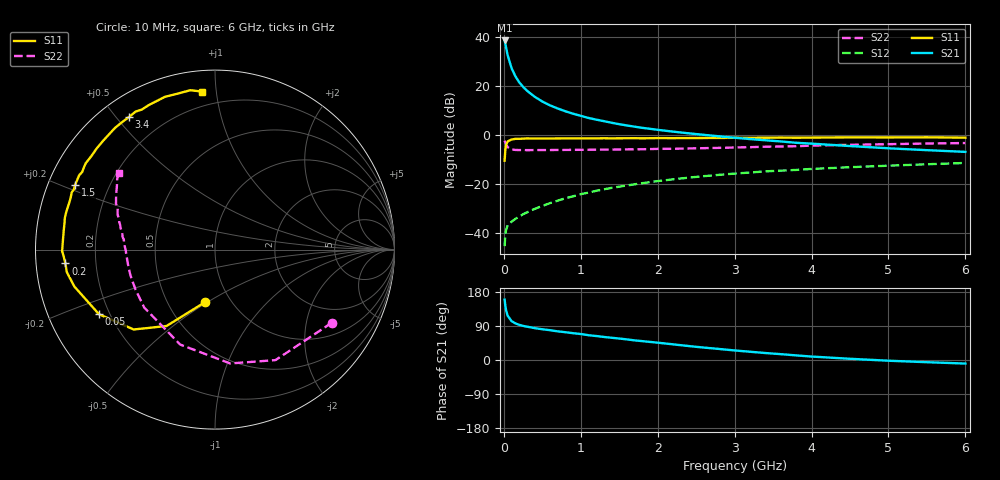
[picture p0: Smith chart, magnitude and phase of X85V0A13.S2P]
! SIEMENS Small Signal Semiconductors
! BFP136W
! Si NPN RF Bipolar Junction Transistor in SOT343
! VCE = 5 V  IC = 130 mA
! Common Emitter S-Parameters:  September  1994
# GHz  S  MA  R  50
!  f  S11  S21  S12  S22
! GHz  MAG  ANG  MAG  ANG  MAG  ANG  MAG  ANG
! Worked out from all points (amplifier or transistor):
!   40 points, 10 MHz to 6 GHz, reference 50 ohm
!   highest |S21| = 38.7 dB at 10 MHz (marker M1)
!   |S21| within 3 dB of that: start of sweep to 29.86 MHz
!   unconditionally stable (mu >= 1): 495.4 MHz to 2.976 GHz
!   at 200 MHz: K = 0.71, MSG = 27.5 dB, |S12| = -33.4 dB
!   at 1.5 GHz: K = 1.10, MAG = 10.9 dB, |S12| = -21.1 dB
!   at 6 GHz: K = 0.97, MSG = 2.3 dB, |S12| = -11.4 dB
!   S11 on the Smith chart (normalised r, x): 10 MHz: 0.76, -0.49; 50 MHz: 0.16, -0.25; 200 MHz: 0.09, -0.05; 1.5 GHz: 0.08, +0.22; 3.4 GHz: 0.08, +0.54; 6 GHz: 0.11, +0.91
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0.01  0.2988 -100.9  86.44 159.3  0.0053 67.9  0.7682 -32.0
0.02  0.5042 -122.4  73.26 142.2  0.0094 54.5  0.7019 -61.3
0.03  0.6351 -135.5  61.04 130.4  0.0115 48.6  0.64 -82.4
0.05  0.74 -150.9  42.98 116.6  0.0142 38.1  0.5635 -110.1
0.1  0.8102 -165.3  23.55 102.7  0.0168 37.5  0.5097 -140.7
0.15  0.8353 -171.4  15.98 96.6  0.0192 40.6  0.4956 -153.2
0.2  0.8368 -174.7  12.01 92.8  0.0215 42.7  0.4925 -159.8
0.25  0.8446 -177.6  9.676 90.0  0.0239 45.9  0.4922 -164.2
0.3  0.8518 -179.4  8.094 88.0  0.0261 48.4  0.4909 -167.0
0.4  0.849 177.0  6.098 84.2  0.0307 52.8  0.4919 -170.9
0.5  0.8488 174.3  4.859 81.1  0.0353 55.5  0.4926 -173.6
0.6  0.8498 172.3  4.055 78.7  0.0403 57.5  0.4933 -175.4
0.7  0.8517 169.8  3.496 75.6  0.0453 59.4  0.495 -176.7
0.9  0.8547 166.2  2.735 70.8  0.0557 60.6  0.4968 -179.2
1.1  0.8531 161.9  2.238 65.4  0.0663 61.2  0.5001 179.2
1.5  0.8585 155.3  1.667 56.6  0.0877 60.3  0.5056 176.0
2.2  0.8637 142.9  1.174 41.3  0.1238 55.2  0.523 170.6
3.2  0.8788 126.1  0.827 21.8  0.1708 45.5  0.5643 161.9
3.4  0.8804 123.0  0.782 18.4  0.1804 43.5  0.5767 160.2
4.5  0.8957 108.1  0.595 3.2  0.2195 33.6  0.6309 150.8
5.5  0.8987 98.8  0.49 -5.8  0.2521 25.5  0.6705 144.4
6  0.8832 94.7  0.452 -9.4  0.2681 21.2  0.6861 141.5
